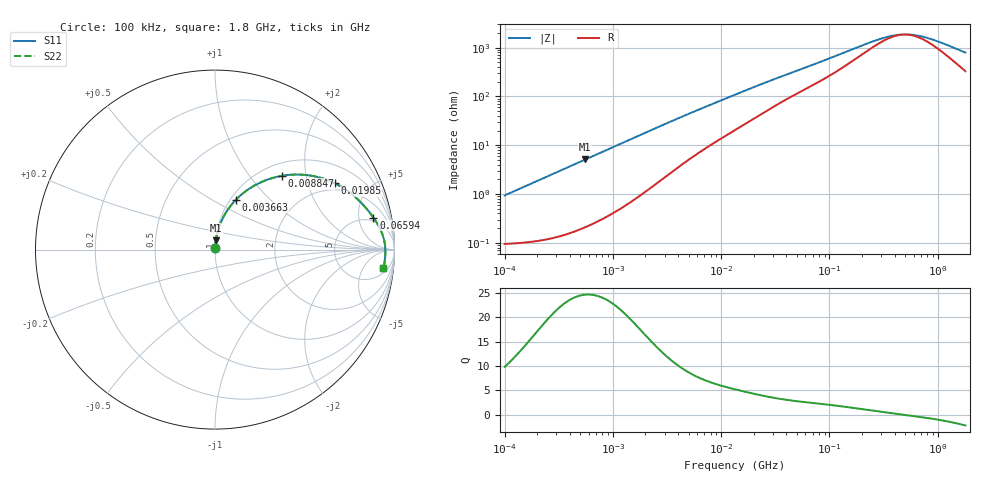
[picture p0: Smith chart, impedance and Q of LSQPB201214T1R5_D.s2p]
! LSQPB201214T1R5_D  S-PARAMETER MODEL  ( General Type )
! Model Generated by TAIYO YUDEN Corporation (http://www.ty-top.com)
! Version 1.0
! TAIYO YUDEN Control No. 100901NG22SB-FKC
! Copyright(c) 2010 TAIYO YUDEN CO.,LTD. All Rights Reserved.
! Product Description (link to TY-COMPAS)
! https://ds.yuden.co.jp/TYCOMPAS/or/detail?pn=LSQPB201214T1R5MD&u=M
! Products Name : Inductors
! Characteristics :
!  Inductance : 1.5 uH , SRF(min) : 390 MHz , DC Resistance(max) : 0.117 Ohm
!  Rated Current : Saturation :1200 mA , Temp Rise : 1100 mA (40 degC)
!  Case Size : 2.0 x 1.25 / 0.079 x 0.049 [mm/inch] , Thickness : 1.4 / 0.056 [mm/inch]
!  (Conditions: Temperature = 25 degC , DC Bias Current/Voltage = 0A / 0V)
! External Node Assignments :
!  1  o---GGG---o  2
! GND o---------o GND
! Frequency Range : 0.1MHz  -  1800MHz  [ 402 STEP ]
# MHz S RI R 50
! Freq[MHz].  S11 Real  S11 Imag  S21 Real  S21 Imag  S12 Real  S12 Imag  S22 Real  S22 Imag
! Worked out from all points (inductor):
!   401 points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, 100 kHz to 1.8 GHz, reference 50 ohm
!   read as one part in series: L = 1.48 uH near 105 kHz
!   highest Q = 24.6 at 555.5 kHz (marker M1), where L = 1.47 uH
!   self-resonance near 491.4 MHz
!   S11 on the Smith chart (normalised r, x): 100 kHz: 1.00, +0.02; 3.663 MHz: 1.06, +0.65; 8.847 MHz: 1.23, +1.47; 19.85 MHz: 1.69, +3.00; 65.94 MHz: 4.16, +7.84; 1.8 GHz: 8, -14
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0.1  0.00103 0.00928  0.999 -0.00928  0.999 -0.00928  0.00103 0.00928
0.516129  0.00419 0.0474  0.9958 -0.0474  0.9958 -0.0474  0.00419 0.0474
0.555485  0.00468 0.0509  0.9953 -0.0509  0.9953 -0.0509  0.00468 0.0509
1.277529  0.0188 0.1139  0.9812 -0.1139  0.9812 -0.1139  0.0188 0.1139
2.66389  0.0692 0.2193  0.9308 -0.2193  0.9308 -0.2193  0.0692 0.2193
3.662795  0.1176 0.2788  0.8824 -0.2788  0.8824 -0.2788  0.1176 0.2788
5.554714  0.2172 0.3555  0.7828 -0.3555  0.7828 -0.3555  0.2172 0.3555
8.84682  0.3747 0.4114  0.6253 -0.4114  0.6253 -0.4114  0.3747 0.4114
13.41641  0.534 0.4121  0.466 -0.4121  0.466 -0.4121  0.534 0.4121
19.85396  0.6686 0.3691  0.3314 -0.3691  0.3314 -0.3691  0.6686 0.3691
25.99364  0.7413 0.3251  0.2587 -0.3251  0.2587 -0.3251  0.7413 0.3251
34.03197  0.797 0.2784  0.203 -0.2784  0.203 -0.2784  0.797 0.2784
65.93531  0.8829 0.1779  0.1171 -0.1779  0.1171 -0.1779  0.8829 0.1779
69.24595  0.8873 0.1715  0.1127 -0.1715  0.1127 -0.1715  0.8873 0.1715
121.6389  0.9245 0.1059  0.0755 -0.1059  0.0755 -0.1059  0.9245 0.1059
241.5136  0.9438 0.0461  0.0562 -0.0461  0.0562 -0.0461  0.9438 0.0461
357.3983  0.9477 0.0196  0.0523 -0.0196  0.0523 -0.0196  0.9477 0.0196
491.4156  0.949 -2.67e-06  0.051 2.67e-06  0.051 2.67e-06  0.949 -2.67e-06
569.2172  0.9492 -0.009  0.0508 0.009  0.0508 0.009  0.9492 -0.009
675.6865  0.9491 -0.0198  0.0509 0.0198  0.0509 0.0198  0.9491 -0.0198
975.7037  0.9476 -0.0452  0.0524 0.0452  0.0524 0.0452  0.9476 -0.0452
1800  0.9387 -0.1026  0.0613 0.1026  0.0613 0.1026  0.9387 -0.1026
